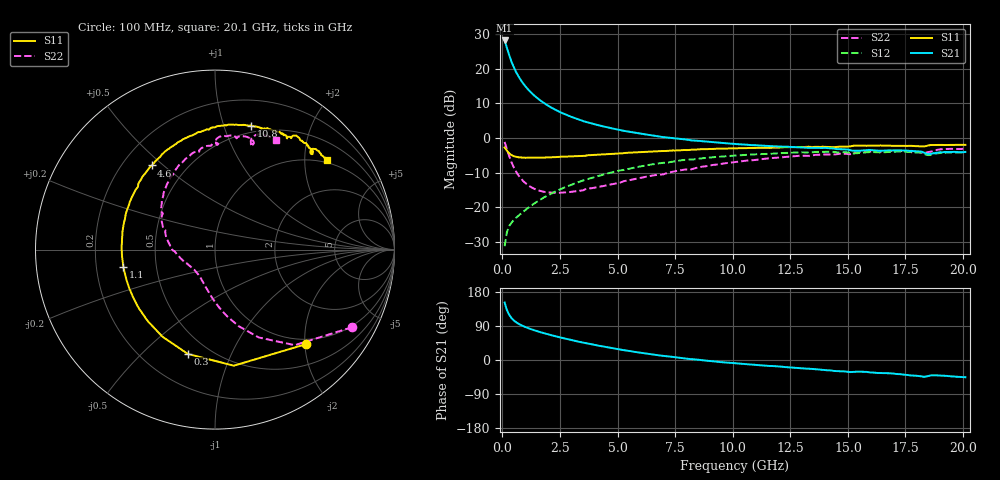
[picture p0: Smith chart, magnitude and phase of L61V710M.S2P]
!  Infineon Technologies AG
! BFR380L3 , PF131585-7, No.6, Th 09.10.01, soldered on pcb-board, measured with PP GSG850
!  Vce=1.75 V,  Ic=10.0 mA
! Common Emitter S-Parameters:  15. November 2001
#  GHz  S  MA  R  50
! f  S11  S21  S12  S22
! GHz  Mag  Ang  Mag  Ang  Mag  Ang  Mag  Ang
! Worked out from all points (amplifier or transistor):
!   201 points, 100 MHz to 20.1 GHz, reference 50 ohm
!   highest |S21| = 28.2 dB at 100 MHz (marker M1)
!   |S21| within 3 dB of that: start of sweep to 241 MHz
!   unconditionally stable (mu >= 1): 1.795 GHz to 4.674 GHz
!   at 3.4 GHz: K = 1.03, MAG = 7.8 dB, |S12| = -12.5 dB
!   at 10.1 GHz: K = 0.96, MSG = 1.7 dB, |S12| = -5.1 dB
!   at 20.1 GHz: K = 0.99, MSG = 0.1 dB, |S12| = -4.1 dB
!   S11 on the Smith chart (normalised r, x): 100 MHz: 0.89, -2.02; 300 MHz: 0.38, -0.70; 1.1 GHz: 0.32, -0.09; 4.6 GHz: 0.32, +0.46; 10.8 GHz: 0.44, +1.24; 20.1 GHz: 0.93, +2.55
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0.1  0.7311 -46.1  25.59 151.5  0.02752 68.4  0.8775 -29.5
0.2  0.6552 -80.8  20.02 131.6  0.04406 56.3  0.6933 -50.2
0.3  0.6008 -104.6  15.69 119.1  0.05391 50.3  0.5469 -63.5
0.4  0.5666 -121.1  12.64 110.5  0.06014 48.1  0.4458 -72.9
0.5  0.547 -133.1  10.51 104.4  0.06554 48.0  0.3761 -79.9
0.6  0.536 -142.4  8.951 99.7  0.07078 48.3  0.3266 -85.5
0.7  0.5278 -149.9  7.792 95.8  0.07573 49.3  0.29 -90.3
0.8  0.524 -155.7  6.886 92.5  0.08097 50.3  0.2621 -94.5
0.9  0.5216 -160.8  6.168 89.6  0.08629 51.3  0.2406 -98.2
1.1  0.5196 -169.1  5.115 84.6  0.09726 53.0  0.2112 -105.0
1.3  0.5192 -175.7  4.364 80.2  0.1085 54.3  0.1914 -110.8
1.5  0.5211 178.5  3.814 76.2  0.1201 55.3  0.1788 -116.1
2  0.5263 167.1  2.913 67.5  0.1503 56.2  0.1643 -127.8
2.6  0.5377 155.8  2.293 58.3  0.1875 55.4  0.1632 -139.8
3.5  0.554 141.6  1.762 46.0  0.244 52.2  0.1758 -154.1
4.6  0.5867 127.0  1.416 33.1  0.3109 46.6  0.2106 -171.5
6.8  0.6466 103.2  1.056 12.2  0.4313 32.6  0.296 159.6
10.1  0.7092 78.0  0.8222 -8.5  0.5576 11.2  0.4505 126.6
10.8  0.7189 73.6  0.7901 -11.9  0.5763 6.7  0.4772 119.6
13.5  0.7431 60.2  0.7227 -23.9  0.6246 -9.7  0.5646 98.4
16.8  0.7768 47.9  0.6645 -35.1  0.6292 -25.6  0.6478 77.1
20.1  0.7971 38.7  0.6297 -45.4  0.6209 -39.2  0.6986 60.9
